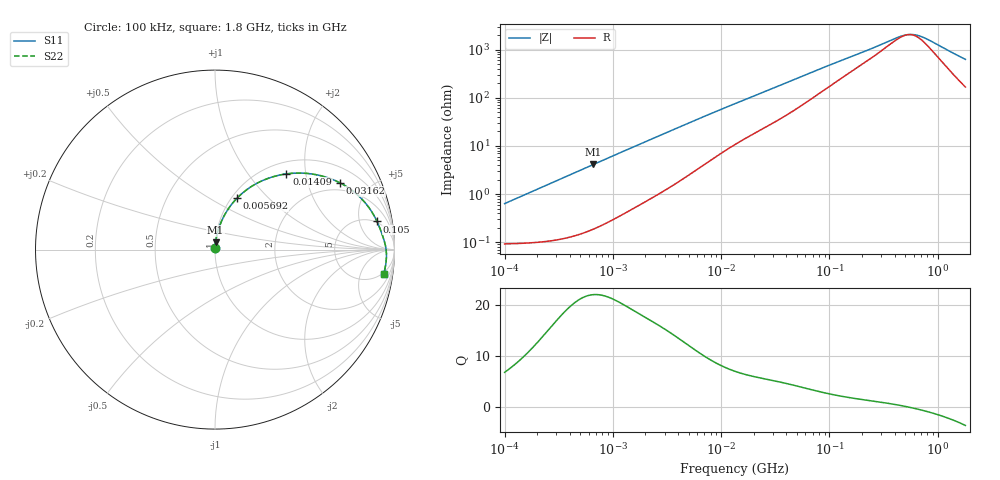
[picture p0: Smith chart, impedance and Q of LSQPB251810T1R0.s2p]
! LSQPB251810T1R0  S-PARAMETER MODEL  ( General Type )
! Model Generated by TAIYO YUDEN Corporation (http://www.ty-top.com)
! Version 2.0
! TAIYO YUDEN Control No. 100810NG22EB-FKC
! Copyright(c) 2009 TAIYO YUDEN CO.,LTD. All Rights Reserved.
! Product Description (link to TY-COMPAS)
! https://ds.yuden.co.jp/TYCOMPAS/or/detail?pn=LSQPB251810T1R0M&u=M
! Products Name : Inductors
! Characteristics :
!  Inductance : 1.0 uH , SRF(min) : 130 MHz , DC Resistance(max) : 0.117 Ohm
!  Rated Current : Saturation :1200 mA , Temp Rise : 1200 mA (40 degC)
!  Case Size : 2.5 x 1.8 / 0.098 x 0.071 [mm/inch] , Thickness : 1.0 / 0.04 [mm/inch]
!  (Conditions: Temperature = 25 degC , DC Bias Current/Voltage = 0A / 0V)
! External Node Assignments :
!  1  o---GGG---o  2
! GND o---------o GND
! Frequency Range : 0.1MHz  -  1800MHz  [ 402 STEP ]
# MHz S RI R 50
! Freq[MHz].  S11 Real  S11 Imag  S21 Real  S21 Imag  S12 Real  S12 Imag  S22 Real  S22 Imag
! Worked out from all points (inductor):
!   401 points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, 100 kHz to 1.8 GHz, reference 50 ohm
!   read as one part in series: L = 1 uH near 105 kHz
!   highest Q = 22 at 659.4 kHz (marker M1), where L = 994 nH
!   self-resonance near 533 MHz
!   S11 on the Smith chart (normalised r, x): 100 kHz: 1.00, +0.01; 5.692 MHz: 1.06, +0.67; 14.09 MHz: 1.23, +1.56; 31.62 MHz: 1.64, +3.23; 105 MHz: 5, +9; 1.8 GHz: 4, -12
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0.1  0.000963 0.00627  0.999 -0.00627  0.999 -0.00627  0.000963 0.00627
0.516129  0.00255 0.0322  0.9975 -0.0322  0.9975 -0.0322  0.00255 0.0322
0.659386  0.00355 0.041  0.9964 -0.041  0.9964 -0.041  0.00355 0.041
1.409041  0.0118 0.0855  0.9882 -0.0855  0.9882 -0.0855  0.0118 0.0855
2.66389  0.0346 0.1543  0.9654 -0.1543  0.9654 -0.1543  0.0346 0.1543
4.039851  0.0701 0.2208  0.9299 -0.2208  0.9299 -0.2208  0.0701 0.2208
5.692459  0.1226 0.2865  0.8774 -0.2865  0.8774 -0.2865  0.1226 0.2865
8.423854  0.2185 0.3611  0.7815 -0.3611  0.7815 -0.3611  0.2185 0.3611
13.41641  0.3792 0.4189  0.6208 -0.4189  0.6208 -0.4189  0.3792 0.4189
14.09005  0.398 0.4218  0.602 -0.4218  0.602 -0.4218  0.398 0.4218
20.85084  0.5507 0.4196  0.4493 -0.4196  0.4493 -0.4196  0.5507 0.4196
31.62078  0.6972 0.3716  0.3028 -0.3716  0.3028 -0.3716  0.6972 0.3716
46.79328  0.7999 0.2996  0.2001 -0.2996  0.2001 -0.2996  0.7999 0.2996
69.24595  0.8646 0.2242  0.1354 -0.2242  0.1354 -0.2242  0.8646 0.2242
105.0131  0.9027 0.1566  0.0973 -0.1566  0.0973 -0.1566  0.9027 0.1566
218.9722  0.9347 0.0744  0.0653 -0.0744  0.0653 -0.0744  0.9347 0.0744
357.3983  0.9471 0.0332  0.0529 -0.0332  0.0529 -0.0332  0.9471 0.0332
503.6016  0.9527 0.00484  0.0473 -0.00484  0.0473 -0.00484  0.9527 0.00484
569.2172  0.954 -0.00571  0.046 0.00571  0.046 0.00571  0.954 -0.00571
643.382  0.9548 -0.0166  0.0452 0.0166  0.0452 0.0166  0.9548 -0.0166
802.0705  0.9552 -0.0375  0.0448 0.0375  0.0448 0.0375  0.9552 -0.0375
1800  0.9388 -0.1385  0.0612 0.1385  0.0612 0.1385  0.9388 -0.1385
